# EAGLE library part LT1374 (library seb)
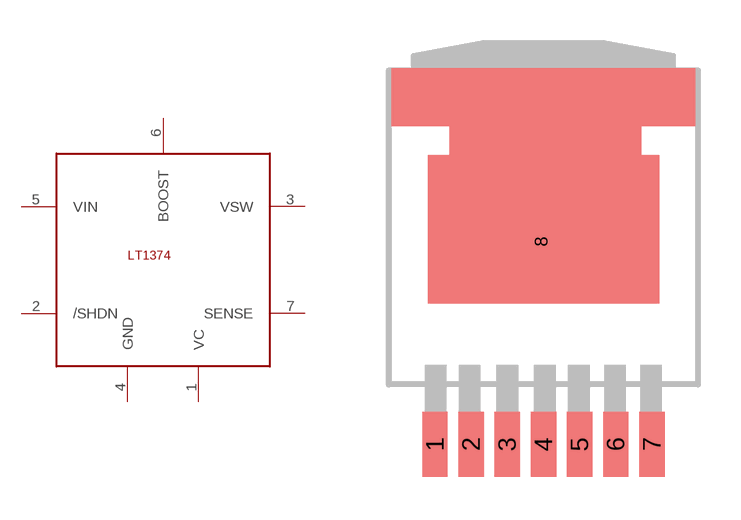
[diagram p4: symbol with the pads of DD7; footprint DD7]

Designator prefix IC

## LT1374  [DD7]
1  VC
2  /SHDN
3  VSW
4  GND
5  VIN
6  BOOST
7  SENSE

## Footprint DD7 (pad centres in mm)
smd 0.889 x 2.286: 1 -3.81,-7.112; 2 -2.54,-7.112; 3 -1.27,-7.112; 4 0,-7.112; 5 1.27,-7.112; 6 2.54,-7.112; 7 3.81,-7.112
smd 0.635 x 2.286: 8 -0.071,0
